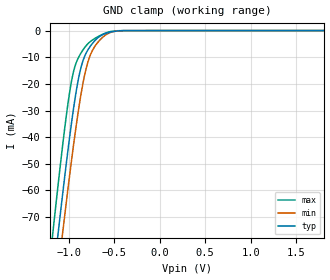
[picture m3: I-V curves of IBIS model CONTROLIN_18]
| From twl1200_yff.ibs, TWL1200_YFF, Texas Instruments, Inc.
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[Model]   CONTROLIN_18
Model_type  Input
Vinl=0.63
Vinh=1.17
| variable   typ   min   max
C_comp   1.91pF   1.58pF   2.47pF
[Temperature Range]   40   100   -40
| Ambient temperature   25   85   -40
[Voltage range]   1.8   1.65   1.95
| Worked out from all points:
|   GND clamp passes 1 mA (typ) near -0.59 V on its own axis
[GND Clamp]
| CONTROLIN_18
|   Voltage   I(typ)   I(min)   I(max)
-1.8V     -299.4mA   -308.8mA   -288.2mA
-1.18V    -96.35mA   -110.5mA   -78.5mA
-1.16V    -90.16mA   -104.4mA   -72.15mA
-1.115V   -76.42mA   -90.86mA   -58.14mA
-1.06V    -60.12mA   -74.69mA   -41.82mA
-965mV    -34.16mA   -48.22mA   -18.62mA
-880mV    -16.32mA   -27.48mA   -9.428mA
-795mV    -7.709mA   -12.73mA   -5.221mA
-705mV    -3.573mA   -5.62mA    -2.835mA
-585mV    -997.9uA   -1.471mA   -816.9uA
-435mV    -81.06uA   -95.31uA   -26.16uA
1.8V      127.8pA    817pA      24.46pA
